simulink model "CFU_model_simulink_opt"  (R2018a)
settings: Solver=ode15s  StartTime=0.0  StopTime=30000  RelTol=1e-6
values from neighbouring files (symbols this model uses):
  D_val = [F_in; ppm_in]    [Casadi_model.m]
  gain_float = [0 1]    [OL_CL_PID.m]
  gain_outflow = [0 1]    [OL_CL_PID.m]
  gain_reject = [0 1]    [OL_CL_PID.m]
  t_float = 16000    [OL_CL_PID.m]
  t_out = 10000    [OL_CL_PID.m]
  t_reject = 15000    [OL_CL_PID.m]
  U_val = x0_IPOPT(36:38)    [Casadi_model.m]
  x0 = x0_IPOPT(1:35)    [Casadi_model.m]    (also in OL_CL_PID.m = x_initial)
undefined symbols (not defined in the file or in its folder): CFU_model_sim
libraries: simulink x3

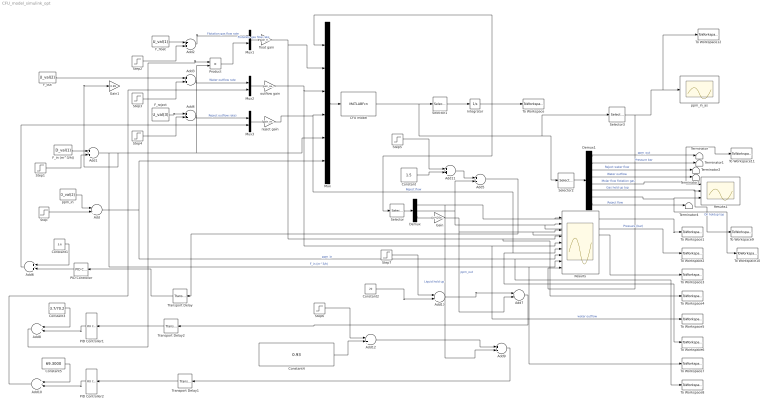
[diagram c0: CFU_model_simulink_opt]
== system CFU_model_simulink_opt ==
  Add{,1..4,6,8,10..13} (11 alike) : Sum
  Add5 : Sum  Inputs=+-
  Add7 : Sum  Inputs=+-
  Add9 : Sum  Inputs=+-
  CFU model : MATLABFcn  MATLABFcn=CFU_model_sim(u(1:35),u(36:38),u(39:40))
  Constant : Constant  Value=1.5
  Constant1 : Constant  Value=5.6
  Constant2 : Constant  Value=20
  Constant3 : Constant  Value=3.7/70.2
  Constant4 : Constant  Value=0.93
  Constant5 : Constant  Value=69.3000
  Demux : Demux  Outputs=3
  Demux1 : Demux  Outputs=8
  F_float : Constant  Value=U_val(1)
  F_in (m^3/h)) : Constant  Value=D_val(1)
  F_out : Constant  Value=U_val(2)
  F_reject : Constant  Value=U_val(3)
  Gain : Gain  Gain=pi*(25e-6)^3/6 * 1e10*1e6
  Gain1 : Gain  Commented=on  Gain=0.99
  Integrator : Integrator  InitialCondition=x0
  Mux : Mux  Inputs=6
  Mux1 : Mux  Inputs=2
  Mux2 : Mux  Inputs=2
  Mux3 : Mux  Inputs=2
  PID Controller : simulink/Continuous/PID Controller  Controller=PI  TimeDomain=Continuous-time  SampleTime=-1  IntegratorMethod=Forward Euler  FilterMethod=Forward Euler  Form=Ideal  UseFilter=on  ControllerParametersSource=internal  P=-55.75  I=1/200  D=0  N=100  InitialConditionSource=internal  InitialConditionForIntegrator=0  InitialConditionForFilter=0  ExternalReset=none  LimitOutput=off  UpperSaturationLimit=inf  LowerSaturationLimit=0  LinearizeAsGain=on  AntiWindupMode=clamping  Kb=1  TrackingMode=off  Kt=1  PParamMin=[]  PParamMax=[]  IParamMin=[]  IParamMax=[]  DParamMin=[]  DParamMax=[]  NParamMin=[]  NParamMax=[]  KbParamMin=[]  KbParamMax=[]  KtParamMin=[]  KtParamMax=[]  POutMin=[]  POutMax=[]  IOutMin=[]  IOutMax=[]  DOutMin=[]  DOutMax=[]  NOutMin=[]  NOutMax=[]  KbOutMin=[]  KbOutMax=[]  KtOutMin=[]  KtOutMax=[]  IntegratorOutMin=[]  IntegratorOutMax=[]  FilterOutMin=[]  FilterOutMax=[]  SumOutMin=[]  SumOutMax=[]  SumI1OutMin=[]  SumI1OutMax=[]  SumI2OutMin=[]  SumI2OutMax=[]  SumI3OutMin=[]  SumI3OutMax=[]  SumDOutMin=[]  SumDOutMax=[]  SaturationOutMin=[]  SaturationOutMax=[]  IntegratorContinuousStateAttributes=''  IntegratorStateMustResolveToSignalObject=off  IntegratorRTWStateStorageClass=Auto  FilterContinuousStateAttributes=''  FilterStateMustResolveToSignalObject=off  FilterRTWStateStorageClass=Auto  DifferentiatorICPrevScaledInput=0  DifferentiatorOutMin=[]  DifferentiatorOutMax=[]  InitialConditionSetting=State (most efficient)  FilterDiffOutCoefMin=[]  FilterDiffOutCoefMax=[]  SumDenOutMin=[]  SumDenOutMax=[]  SumNumOutMin=[]  SumNumOutMax=[]  ReciprocalOutMin=[]  ReciprocalOutMax=[]  DivideOutMin=[]  DivideOutMax=[]  TunerSelectOption=Transfer Function Based (PID Tuner App)
  PID Controller1 : simulink/Continuous/PID Controller  Controller=PI  TimeDomain=Continuous-time  SampleTime=-1  IntegratorMethod=Forward Euler  FilterMethod=Forward Euler  Form=Ideal  UseFilter=on  ControllerParametersSource=internal  P=-0.25/70.2  I=1/316  D=0  N=100  InitialConditionSource=internal  InitialConditionForIntegrator=0  InitialConditionForFilter=0  ExternalReset=none  LimitOutput=off  UpperSaturationLimit=inf  LowerSaturationLimit=-inf  LinearizeAsGain=on  AntiWindupMode=none  Kb=1  TrackingMode=off  Kt=1  PParamMin=[]  PParamMax=[]  IParamMin=[]  IParamMax=[]  DParamMin=[]  DParamMax=[]  NParamMin=[]  NParamMax=[]  KbParamMin=[]  KbParamMax=[]  KtParamMin=[]  KtParamMax=[]  POutMin=[]  POutMax=[]  IOutMin=[]  IOutMax=[]  DOutMin=[]  DOutMax=[]  NOutMin=[]  NOutMax=[]  KbOutMin=[]  KbOutMax=[]  KtOutMin=[]  KtOutMax=[]  IntegratorOutMin=[]  IntegratorOutMax=[]  FilterOutMin=[]  FilterOutMax=[]  SumOutMin=[]  SumOutMax=[]  SumI1OutMin=[]  SumI1OutMax=[]  SumI2OutMin=[]  SumI2OutMax=[]  SumI3OutMin=[]  SumI3OutMax=[]  SumDOutMin=[]  SumDOutMax=[]  SaturationOutMin=[]  SaturationOutMax=[]  IntegratorContinuousStateAttributes=''  IntegratorStateMustResolveToSignalObject=off  IntegratorRTWStateStorageClass=Auto  FilterContinuousStateAttributes=''  FilterStateMustResolveToSignalObject=off  FilterRTWStateStorageClass=Auto  DifferentiatorICPrevScaledInput=0  DifferentiatorOutMin=[]  DifferentiatorOutMax=[]  InitialConditionSetting=State (most efficient)  FilterDiffOutCoefMin=[]  FilterDiffOutCoefMax=[]  SumDenOutMin=[]  SumDenOutMax=[]  SumNumOutMin=[]  SumNumOutMax=[]  ReciprocalOutMin=[]  ReciprocalOutMax=[]  DivideOutMin=[]  DivideOutMax=[]  TunerSelectOption=Transfer Function Based (PID Tuner App)
  PID Controller2 : simulink/Continuous/PID Controller  Controller=PI  TimeDomain=Continuous-time  SampleTime=-1  IntegratorMethod=Forward Euler  FilterMethod=Forward Euler  Form=Ideal  UseFilter=on  ControllerParametersSource=internal  P=-318.19  I=1/204  D=0  N=100  InitialConditionSource=internal  InitialConditionForIntegrator=0  InitialConditionForFilter=0  ExternalReset=none  LimitOutput=off  UpperSaturationLimit=inf  LowerSaturationLimit=-inf  LinearizeAsGain=on  AntiWindupMode=none  Kb=1  TrackingMode=off  Kt=1  PParamMin=[]  PParamMax=[]  IParamMin=[]  IParamMax=[]  DParamMin=[]  DParamMax=[]  NParamMin=[]  NParamMax=[]  KbParamMin=[]  KbParamMax=[]  KtParamMin=[]  KtParamMax=[]  POutMin=[]  POutMax=[]  IOutMin=[]  IOutMax=[]  DOutMin=[]  DOutMax=[]  NOutMin=[]  NOutMax=[]  KbOutMin=[]  KbOutMax=[]  KtOutMin=[]  KtOutMax=[]  IntegratorOutMin=[]  IntegratorOutMax=[]  FilterOutMin=[]  FilterOutMax=[]  SumOutMin=[]  SumOutMax=[]  SumI1OutMin=[]  SumI1OutMax=[]  SumI2OutMin=[]  SumI2OutMax=[]  SumI3OutMin=[]  SumI3OutMax=[]  SumDOutMin=[]  SumDOutMax=[]  SaturationOutMin=[]  SaturationOutMax=[]  IntegratorContinuousStateAttributes=''  IntegratorStateMustResolveToSignalObject=off  IntegratorRTWStateStorageClass=Auto  FilterContinuousStateAttributes=''  FilterStateMustResolveToSignalObject=off  FilterRTWStateStorageClass=Auto  DifferentiatorICPrevScaledInput=0  DifferentiatorOutMin=[]  DifferentiatorOutMax=[]  InitialConditionSetting=State (most efficient)  FilterDiffOutCoefMin=[]  FilterDiffOutCoefMax=[]  SumDenOutMin=[]  SumDenOutMax=[]  SumNumOutMin=[]  SumNumOutMax=[]  ReciprocalOutMin=[]  ReciprocalOutMax=[]  DivideOutMin=[]  DivideOutMax=[]  TunerSelectOption=Transfer Function Based (PID Tuner App)
  Product : Product
  Results : Scope  NumInputPorts=9
  Results1 : Scope  NumInputPorts=3
  Selector : Selector  InputPortWidth=35  IndexOptions=Index vector (dialog)  Indices=[31 32 33]  OutputSizes=1
  Selector1 : Selector  InputPortWidth=44  IndexOptions=Index vector (dialog)  Indices=[1:35]  OutputSizes=1
  Selector2 : Selector  InputPortWidth=44  IndexOptions=Index vector (dialog)  Indices=[37:44]  OutputSizes=1
  Selector3 : Selector  InputPortWidth=44  IndexOptions=Index vector (dialog)  Indices=[36]  OutputSizes=1
  Step : Step  Time=25000  After=20  SampleTime=0
  Step1 : Step  Time=20000  After=10  SampleTime=0
  Step2 : Step  Time=t_float  After=0.1  SampleTime=0
  Step3 : Step  Time=t_out  After=0.9  SampleTime=0
  Step4 : Step  Time=t_reject  After=0.1  SampleTime=0
  Step5 : Step  Time=5000  After=-0.03  SampleTime=0
  Step6 : Step  Time=10000  After=-0.03  SampleTime=0
  Step7 : Step  Time=15000  After=5  SampleTime=0
  Terminator{,1..4} (5 alike) : Terminator
  To Workspace : ToWorkspace  VariableName=x_simulink  SampleTime=-1
  To Workspace1 : ToWorkspace  VariableName=liq_hold_up  SampleTime=-1
  To Workspace10 : ToWorkspace  VariableName=oil_hold_up  SampleTime=-1
  To Workspace11 : ToWorkspace  VariableName=mass_flow_flotation  SampleTime=-1
  To Workspace12 : ToWorkspace  VariableName=ppm_in_as  SampleTime=-1
  To Workspace2 : ToWorkspace  VariableName=Pressure  SampleTime=-1
  To Workspace3 : ToWorkspace  VariableName=ppm_out  SampleTime=-1
  To Workspace4 : ToWorkspace  VariableName=F_flotation  SampleTime=-1
  To Workspace5 : ToWorkspace  VariableName=F_out  SampleTime=-1
  To Workspace6 : ToWorkspace  VariableName=F_reject  SampleTime=-1
  To Workspace7 : ToWorkspace  VariableName=F_in  SampleTime=-1
  To Workspace8 : ToWorkspace  VariableName=ppm_in  SampleTime=-1
  To Workspace9 : ToWorkspace  VariableName=gas_hold_up  SampleTime=-1
  Transport Delay : TransportDelay
  Transport Delay1 : TransportDelay  DelayTime=2
  Transport Delay2 : TransportDelay  DelayTime=30
  float gain : Gain  Gain=gain_float  Multiplication=Matrix(K*u)
  outflow gain : Gain  Gain=gain_outflow  Multiplication=Matrix(K*u)
  ppm_in : Constant  Value=D_val(2)
  ppm_in_as : Scope
  reject gain : Gain  Gain=gain_reject  Multiplication=Matrix(K*u)
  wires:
  ppm_in/1 -> Add/1
  Step/1 -> Add/2
  F_in (m^3/h))/1 -> Add1/1
  Step1/1 -> Add1/2
  F_float/1 -> Add2/1
  Step2/1 -> Add2/2
  Step3/1 -> Add3/2
  F_reject/1 -> Add4/1
  Step4/1 -> Add4/2
  Add/1 -> Results/7, To Workspace8/1, Mux/6  "ppm_in"
  Add1/1 -> Results/8, To Workspace7/1, Gain1/1, Product/2, Mux/5  "F_in (m^3/h)"
  outflow gain/1 -> Results/5, To Workspace5/1, Mux/3  "water outflow"
  Add4/1 -> Mux3/1  "Reject outflow rate)"
  Mux/1 -> CFU model/1
  CFU model/1 -> Selector3/1, Selector2/1, Selector1/1
  Selector1/1 -> Integrator/1
  Integrator/1 -> To Workspace/1, Selector/1, Mux/1
  Selector/1 -> Demux/1
  Demux/3 -> Gain/1
  Demux/2 -> Add5/2, Results/2, To Workspace2/1  "Pressure (bar)"
  Demux/1 -> Add9/2, To Workspace1/1, Results/1  "Liquid hold up"
  Add2/1 -> Mux1/1  "Flotation gas flow rate"
  Gain/1 -> Results/3, To Workspace3/1, Add7/2  "ppm_out"
  F_out/1 -> Add3/1
  Constant/1 -> Add11/2
  Add5/1 -> Transport Delay/1
  PID Controller/1 -> Add6/2
  Constant1/1 -> Add6/1
  Add6/1 -> Mux3/2
  reject gain/1 -> To Workspace6/1, Results/6, Mux/4  "Reject flow"
  Constant2/1 -> Add13/2
  Add7/1 -> Transport Delay2/1
  Constant3/1 -> Add8/1
  PID Controller1/1 -> Add8/2
  Mux1/1 -> float gain/1  "Flotation gas flow rate"
  Add8/1 -> Product/1
  Selector2/1 -> Demux1/1
  Demux1/1 -> Terminator/1  "ppm_out"
  Demux1/2 -> Terminator1/1  "Pressure bar"
  Demux1/3 -> Terminator2/1  "Reject water flow"
  Demux1/4 -> Terminator3/1  "Water outflow"
  Demux1/5 -> To Workspace11/1, Results1/1  "Molar flow flotation gas"
  Demux1/6 -> To Workspace9/1, Results1/2  "Gas hold up top"
  Demux1/7 -> To Workspace10/1, Results1/3  "Oil holdup top"
  Demux1/8 -> Terminator4/1  "Reject flow"
  Add12/1 -> Add9/1
  Add9/1 -> Transport Delay1/1
  Add10/1 -> Mux2/2
  PID Controller2/1 -> Add10/2
  Constant5/1 -> Add10/1
  Add3/1 -> Mux2/1  "Water outflow rate"
  Add11/1 -> Add5/1
  Step5/1 -> Add11/1
  float gain/1 -> Results/4, To Workspace4/1, Mux/2
  Mux2/1 -> outflow gain/1
  Mux3/1 -> reject gain/1
  Step6/1 -> Add12/1
  Constant4/1 -> Add12/2
  Step7/1 -> Add13/1
  Add13/1 -> Add7/1
  Transport Delay/1 -> PID Controller/1
  Transport Delay1/1 -> PID Controller2/1
  Transport Delay2/1 -> PID Controller1/1
  Product/1 -> Mux1/2
  Selector3/1 -> Results/9, To Workspace12/1, ppm_in_as/1
